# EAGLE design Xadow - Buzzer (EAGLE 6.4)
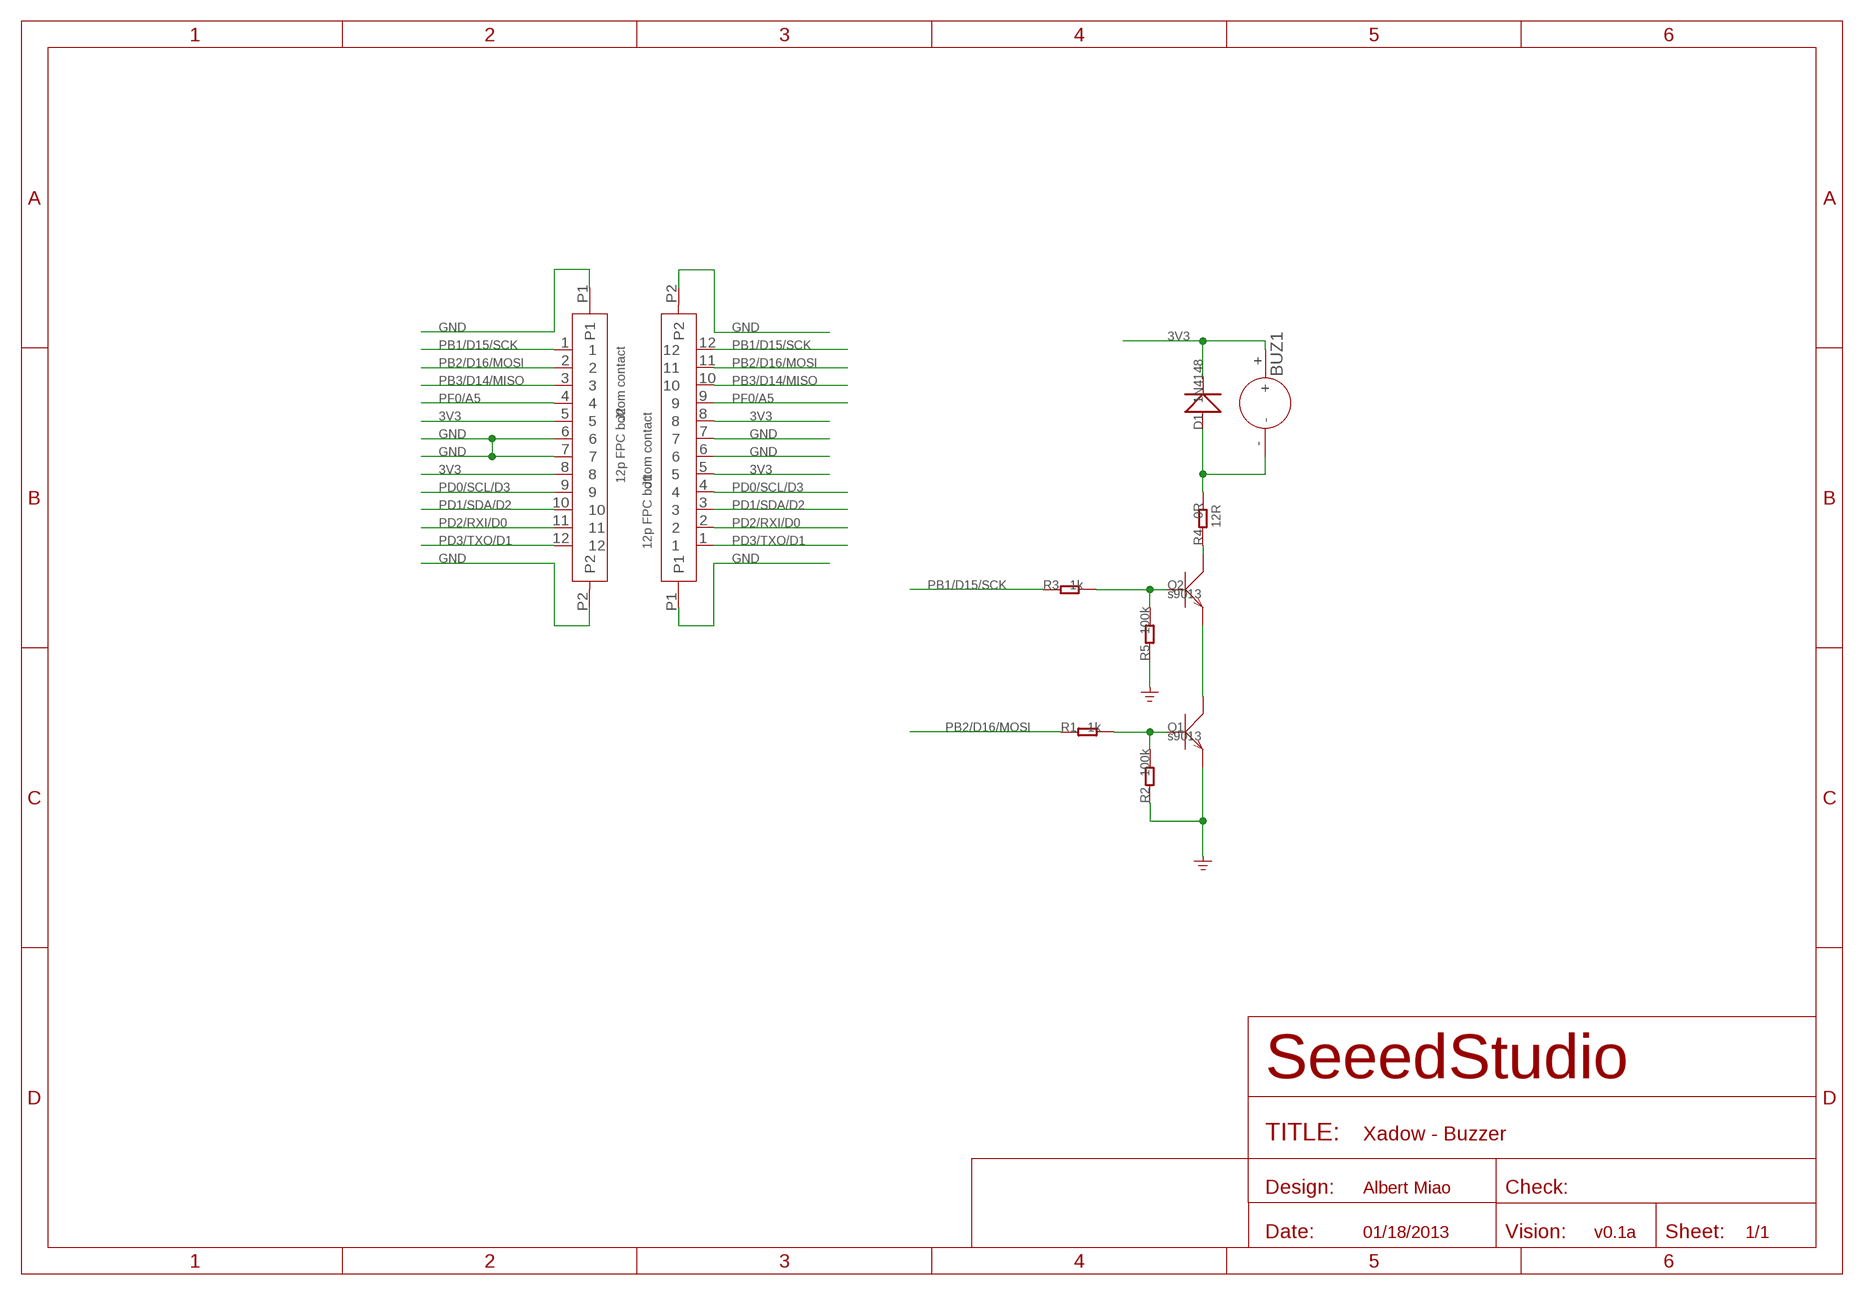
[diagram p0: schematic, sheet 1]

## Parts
BUZ1  BUZZER'KS-SMD-050025'  [3P-5X5X2.5H]
D1  1N4148  D'1206'  [SOD123]
J1  12p FPC bottom contact  FPC052002-12LT  [12P-0.5]
J2  12p FPC bottom contact  FPC052002-12LT  [12P-0.5]
Q1  s9013  TRANSISTOR-NPN-SOT23  [SOT23]
Q2  s9013  TRANSISTOR-NPN-SOT23  [SOT23]
R1  1k  R-0603  [R0603]
R2  100k  R-0603  [R0603]
R3  1k  R-0603  [R0603]
R4  0R  R-0603  [R0603]
R5  100k  R-0603  [R0603]

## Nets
3V3: BUZ1.+ D1.- J1.5 J1.8 J2.5 J2.8
GND: J1.6 J1.7 J1.P1 J1.P2 J2.6 J2.7 J2.P1 J2.P2 Q1.2(E) R2.1 R5.1
N$1: BUZ1.- D1.+ R4.2
N$2: Q1.1(B) R1.2 R2.2
N$3: Q1.3(C) Q2.2(E)
N$5: Q2.3(C) R4.1
N$6: Q2.1(B) R3.2 R5.2
PB1/D15/SCK: J1.12 J2.1 R3.1
PB2/D16/MOSI: J1.11 J2.2 R1.1
PB3/D14/MISO: J1.10 J2.3
PD0/SCL/D3: J1.4 J2.9
PD1/SDA/D2: J1.3 J2.10
PD2/RXI/D0: J1.2 J2.11
PD3/TXO/D1: J1.1 J2.12
PF0/A5: J1.9 J2.4

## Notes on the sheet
- 12R
- Albert Miao
- 01/18/2013 | v0.1a

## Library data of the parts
BUZ1 = template:BUZZER
D1 = Discrete:D*
J1 J2 = template:FPC052002-12LT
Q1 Q2 = Discrete:TRANSISTOR-NPN*: NPN audion
R1-R5 = Discrete:R*

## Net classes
0 default: width 0.152 mm, drill 0.305 mm, clearance 0.152 mm
1 GND: width 0.152 mm, drill 0.305 mm, clearance 0.152 mm to class 0, clearance 0.152 mm
3 usbvcc: width 0.203 mm, drill 0.305 mm, clearance 0.203 mm

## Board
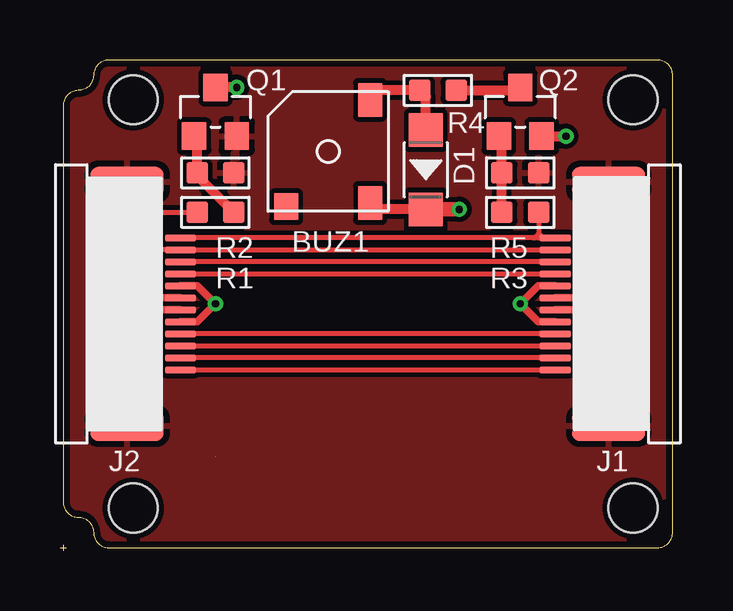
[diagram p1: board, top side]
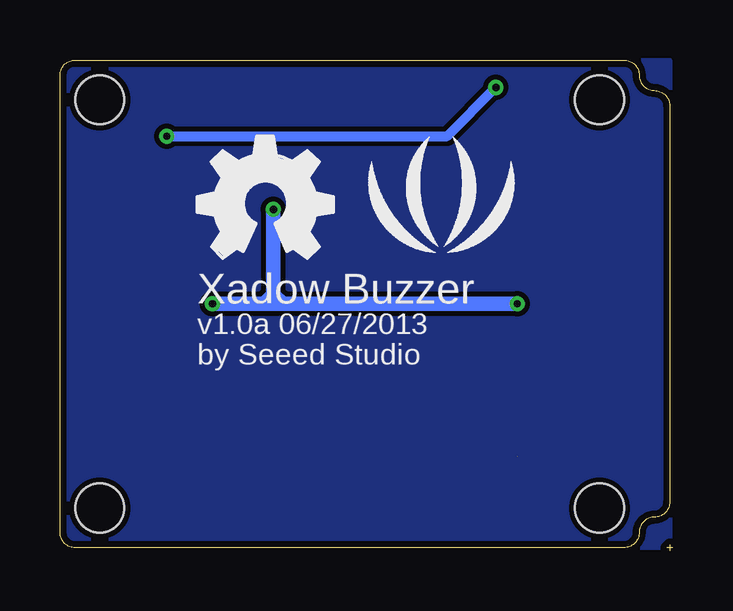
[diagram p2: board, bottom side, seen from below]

Size 25.53 x 20.45 mm. Coordinates in mm from the lower left corner, seen from the top.
Outline: 25.53,19.81 arc90 24.89,20.45
Outline: 2.03,20.45 arc90 1.4,19.81
Outline: 1.4,19.81 arc-90 0.76,19.18
Outline: 0.76,19.18 arc90 0.13,18.54
Outline: 0.13,2.03 arc90 0.76,1.4
Outline: 0.76,1.4 arc-90 1.4,0.76
Outline: 1.4,0.76 arc90 2.03,0.13
Outline: 24.89,0.13 arc90 25.53,0.76
Outline: 25.53,0.76 25.53,19.81
Outline: 25.53,19.81 arc90 24.89,20.45
Outline: 24.89,20.45 2.03,20.45
Outline: 2.03,20.45 arc90 1.4,19.81
Outline: 1.4,19.81 arc-90 0.76,19.18
Outline: 0.76,19.18 arc90 0.13,18.54
Outline: 0.13,18.54 0.13,2.03
Outline: 0.13,2.03 arc90 0.76,1.4
Outline: 0.76,1.4 arc-90 1.4,0.76
Outline: 1.4,0.76 1.4,0.76
Outline: 1.4,0.76 arc90 2.03,0.13
Outline: 2.03,0.13 24.89,0.13
Outline: 24.89,0.13 arc90 25.53,0.76
Outline: 0,0.13 0.25,0.13
Outline: 0.13,0.25 0.13,0
Copper layers (1*16): Top 0.035mm / dielectric 1.5mm / Bottom 0.035mm
Design rules "SeeedStudio_rule_no_angle_090911 *": minimum track width 6mil, minimum drill 12mil, track to track 6mil, track to pad 6mil, pad to pad 6mil, via to via 6mil, smd to smd 0mil, copper to edge 10mil, drill to drill 10mil, minimum pad ring 10mil, minimum via ring 6mil, stop-mask expansion 2mil, vias tented up to drill 25mil, thermal gap 10mil
Holes 2.03 mm at 3.05,1.78 3.05,18.8 23.88,18.8 23.88,1.78
tRestrict: area 20.3,10 to 21,10.5; area 4.8,10 to 5.3,10.5

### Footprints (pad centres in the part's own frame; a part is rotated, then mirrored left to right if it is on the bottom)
3P-5X5X2.5H = smd 1.4 x 1: + -2.15,-1.75; - 2.15,-1.75 | smd 1.1 x 1: NC -2.3,1.75
SOD123 = smd 1.397 x 1.397: + -1.651,0; - 1.651,0
12P-0.5 = smd 0.3 x 1.3: 1 -2.75,2.35; 2 -2.25,2.35; 3 -1.75,2.35; 4 -1.25,2.35; 5 -0.75,2.35; 6 -0.25,2.35; 7 0.25,2.35; 8 0.75,2.35; 9 1.25,2.35; 10 1.75,2.35; 11 2.25,2.35; 12 2.75,2.35 | smd 1.27 x 3.048: P1 -5.08,0.127; P2 5.08,0.127
SOT23 = smd 1.016 x 1.143: 1 -0.889,-1.016; 2 0.889,-1.016; 3 0,1.016
R0603 = smd 0.889 x 0.889: 1 -0.762,0; 2 0.762,0

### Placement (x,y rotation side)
BUZ1  11.18,16.64 90 top
D1  15.24,15.88 270 top
J1  22.99,10.29 90 top
J2  2.67,10.29 270 top
Q1  6.48,18.29 0 top
Q2  19.18,18.29 0 top
R1  6.48,14.1 0 top
R2  6.48,15.75 180 top
R3  19.18,14.1 180 top
R4  15.75,19.18 180 top
R5  19.18,15.75 180 top
U$2  [LOGO_SILK]  9.65,14.1 0 bottom
U$3  [OSHW_FILLX200_NOTEXT]  19.81,12.19 0 bottom

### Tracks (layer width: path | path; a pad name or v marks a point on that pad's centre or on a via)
3V3  (via drill 0.3 pad 0.64)
  Top 0.305: J2.8 5.73,9.54 v6.48,10.29 5.73,11.04 J2.5 | J1.5 19.93,9.54 v19.18,10.29 19.93,11.04 J1.8
  Top 0.406: D1.- 13.19,14.22 BUZ1.+
  Top 0.61: D1.- v16.64,14.22
  Bottom 0.61: v6.48,10.29 16.26,10.29 | 16.51,10.29 17.02,10.29 | 17.02,10.29 v19.18,10.29 | v16.64,14.22 16.64,10.67 | 16.64,10.67 16.64,10.41 16.51,10.29 | 16.64,10.67 17.02,10.29 | 16.64,10.67 16.26,10.29 | 16.26,10.29 16.51,10.29
GND  (1 unrouted)
  Top 0.305: J2.6 3.05,10.54 | J2.7 3.05,10.04 3.05,10.03 | J1.7 22.73,10.54 | J1.6 22.73,10.04 22.73,10.03
  pour Top (isolate 0.203): 0.13,0.13 25.53,0.13 25.53,20.45 0.13,20.45
  pour Bottom (isolate 0.203): 0.13,0.13 25.53,0.13 25.53,20.45 0.13,20.45
N$1
  Top 0.406: BUZ1.- 12.95,18.82 12.95,19.18 R4.2 15.24,18.92 D1.+
N$2
  Top 0.406: Q1.1 5.71,17.14 R2.2 5.71,15.62 R1.2
N$3  (via drill 0.3 pad 0.64)
  Top 0.406: Q2.2 v21.08,17.27 | v7.37,19.3 Q1.3
  Bottom 0.406: v21.08,17.27 9.4,17.27 v7.37,19.3
N$5
  Top 0.406: R4.1 19.05,19.18 Q2.3
N$6
  Top 0.406: R3.2 R5.2 18.41,17.14 Q2.1
PB1/D15/SCK
  Top 0.203: J1.12 19.94,13.04 | 19.94,13.04 19.77,13.04 | J2.1 19.73,13.04 19.77,13.04 | R3.1 19.94,13.21 | 19.94,13.21 19.94,13.04 | 19.94,13.21 20.07,13.08 | 19.77,13.04 19.94,13.21
PB2/D16/MOSI
  Top 0.203: J1.11 J2.2 4.14,12.54 3.94,12.74 3.94,13.92 4.12,14.1 R1.1
PB3/D14/MISO
  Top 0.203: J1.10 J2.3
PD0/SCL/D3
  Top 0.203: J1.4 J2.9
PD1/SDA/D2
  Top 0.203: J2.10 J1.3
PD2/RXI/D0
  Top 0.203: J1.2 J2.11
PD3/TXO/D1
  Top 0.203: J2.12 J1.1
PF0/A5
  Top 0.203: J2.4 J1.9

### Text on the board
bPlace: Xadow Buzzer | v1.0a 06/27/2013 | by Seeed Studio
